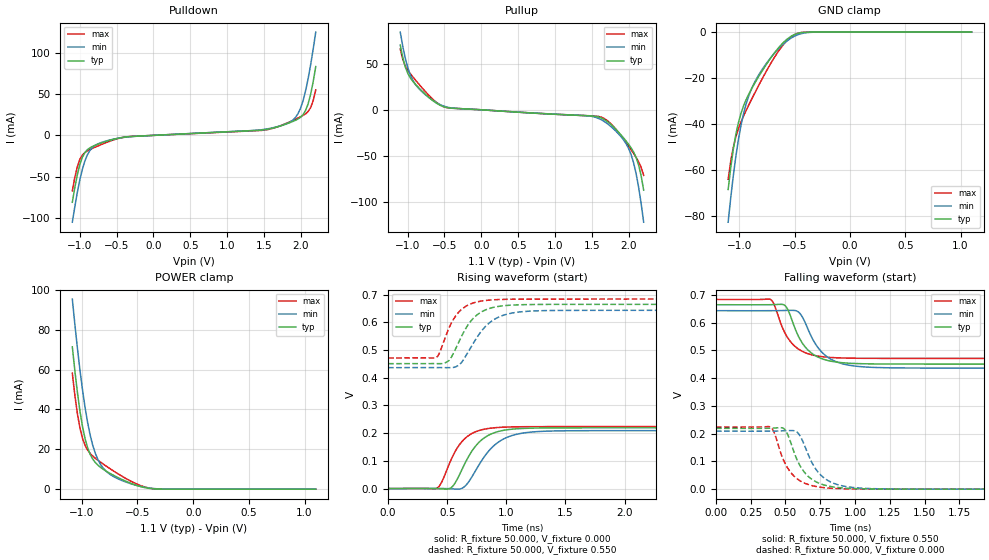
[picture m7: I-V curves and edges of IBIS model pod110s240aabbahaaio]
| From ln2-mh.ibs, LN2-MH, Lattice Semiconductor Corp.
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|   Model pod110s240aabbahaaio
[Model] pod110s240aabbahaaio
| Clamp models do not include dynamic input termination. Please refer to
| the pod110axxxaabbahaain model for input termination.
Model_type I/O
Polarity   Non-Inverting
Enable   Active-Low
Vinl =  0.700V
Vinh =  0.900V
Vmeas =  0.550V
Cref =  20.000pF
Rref =  50.000
Vref =  0.600V
C_comp   2.000pF   1.500pF   2.500pF
[Temperature Range]   25.000   0.125k   -40.000
[Voltage Range]   1.100V   1.070V   1.130V
[C Comp Corner]
C_comp   2.000pF   1.500pF   2.500pF
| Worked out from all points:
|   slope of the pulldown table from 0 to 0.165 V, typ, clamps not added: 226 ohm
|   slope of the pullup table from 0 to 0.165 V, typ, clamps not added: 189 ohm
|   GND clamp passes 1 mA (typ) near -0.50 V on its own axis
|   POWER clamp passes 1 mA (typ) near -0.45 V on its own axis
|   rising waveform, R_fixture 50.000, V_fixture 0.000: 20-80 % time 194ps typ, 223ps min, 170ps max; typ from 0 V to 0.219 V
|   rising waveform, R_fixture 50.000, V_fixture 0.550: 20-80 % time 180ps typ, 213ps min, 152ps max; typ from 0.451 V to 0.665 V
|   falling waveform, R_fixture 50.000, V_fixture 0.550: 20-80 % time 142ps typ, 158ps min, 134ps max; typ from 0.665 V to 0.451 V
|   falling waveform, R_fixture 50.000, V_fixture 0.000: 20-80 % time 136ps typ, 145ps min, 130ps max; typ from 0.219 V to 0 V
[Pulldown]
|Voltage   I(typ)   I(min)   I(max)
-1.1V     -81.17mA   -105.4mA   -67.34mA
-1.032V   -47.86mA   -69.27mA   -37.92mA
-930mV    -20.93mA   -31.09mA   -20.82mA
-862mV    -15.12mA   -18.39mA   -17.27mA
-760mV    -10.94mA   -10.6mA    -13.12mA
-352mV    -1.715mA   -1.886mA   -1.639mA
1.518V    7.039mA    7.489mA    6.6mA
1.892V    16.99mA    18.71mA    18.2mA
1.96V     19.93mA    26.39mA    21.06mA
2.028V    25.15mA    42.13mA    24.19mA
2.13V     49.57mA    85.28mA    33.6mA
2.2V      83.5mA     125.4mA    55.21mA
[Pullup]
|Voltage   I(typ)   I(min)   I(max)
-1.1V     70.38mA    84.41mA    66.13mA
-1.03V    46.02mA    55.41mA    47.25mA
-928mV    30.83mA    31.86mA    35.64mA
-792mV    19.37mA    18.63mA    22.71mA
-554mV    4.731mA    5.428mA    5.061mA
1.452V    -6.529mA   -6.64mA    -6.444mA
1.724V    -13.8mA    -16.09mA   -12.89mA
1.928V    -30.66mA   -32.78mA   -31.94mA
2.03V     -41.41mA   -48.75mA   -43.49mA
2.098V    -51.87mA   -69.53mA   -51.8mA
2.132V    -60.12mA   -84.3mA    -56.57mA
2.2V      -87.31mA   -122.1mA   -71.2mA
[GND_clamp]
|Voltage   I(typ)   I(min)   I(max)
-1.1V     -68.65mA   -82.91mA   -64.16mA
-1.054V   -51.26mA   -62.87mA   -50.37mA
-1.008V   -39.63mA   -47.13mA   -42.26mA
-962mV    -32.34mA   -35.82mA   -36.73mA
-916mV    -27.28mA   -28.13mA   -32.02mA
-847mV    -21.22mA   -20.63mA   -25.4mA
-778mV    -15.81mA   -15.27mA   -19.09mA
-663mV    -7.926mA   -8.201mA   -9.607mA
-571mV    -3.246mA   -3.982mA   -3.828mA
-502mV    -1.097mA   -1.819mA   -1.164mA
-410mV    -96.97uA   -374.9uA   -57.53uA
1.1V      0A         0A         0A
[POWER_clamp]
|Voltage   I(typ)   I(min)   I(max)
-1.085V   71.41mA    95.35mA    58.18mA
-1.062V   59.23mA    82.55mA    46.99mA
-1.039V   48.36mA    70.56mA    37.71mA
-1.016V   38.97mA    59.53mA    30.53mA
-970mV    25.17mA    40.76mA    21.88mA
-924mV    17.37mA    26.93mA    17.87mA
-901mV    15.03mA    21.86mA    16.59mA
-855mV    12.01mA    14.79mA    14.5mA
-763mV    8.448mA    8.108mA    10.89mA
-533mV    2.369mA    2.267mA    3.272mA
-349mV    143.9uA    291.4uA    171.3uA
1.1V      0A         0A         0A
[Ramp]
| variable   typ   min   max
dV/dt_r   0.132/0.194n   0.125/0.224n   0.134/0.171n
dV/dt_f   0.119/0.155n   0.116/0.182n   0.115/0.142n
R_load = 50.000
[Rising Waveform]
R_fixture = 50.000
V_fixture = 0.000
V_fixture_min = 0.000
V_fixture_max = 0.000
|  time   V(typ)   V(min)   V(max)
0s        2.527uV    12.65uV    1.11uV
417ps     24.09uV    252uV      2.484mV
532ps     3.001mV    -643.4uV   103.3mV
621ps     65.34mV    353.3uV    167.8mV
772ps     168.3mV    87.78mV    209.8mV
866ps     195.9mV    142.6mV    217.9mV
962ps     208.9mV    175.6mV    221.3mV
1.157ns   217.3mV    201.4mV    223.2mV
1.507ns   219.1mV    208.5mV    223.6mV
10ns      219.3mV    209.1mV    223.6mV
[Rising Waveform]
R_fixture = 50.000
V_fixture = 0.550
V_fixture_min = 0.534
V_fixture_max = 0.568
|  time   V(typ)   V(min)   V(max)
0s        450.6mV    436.2mV    471.2mV
409ps     450.7mV    436.4mV    473.7mV
510ps     460.3mV    436.2mV    573.9mV
572ps     505mV      439.4mV    623mV
626ps     553.2mV    457.7mV    648mV
722ps     614.9mV    525.2mV    669.9mV
906ps     655.1mV    612.3mV    681.4mV
1.092ns   662.9mV    636.2mV    683.3mV
1.436ns   664.6mV    642.7mV    683.7mV
10ns      664.7mV    643.2mV    683.7mV
[Falling Waveform]
R_fixture = 50.000
V_fixture = 0.550
V_fixture_min = 0.534
V_fixture_max = 0.568
|  time   V(typ)   V(min)   V(max)
0s        664.7mV    643.2mV    683.7mV
392ps     664.8mV    643.2mV    683.7mV
420ps     665.2mV    643.2mV    663.1mV
499ps     660.2mV    644mV      560.1mV
582ps     562.7mV    641.7mV    509mV
651ps     507.1mV    589.2mV    490mV
743ps     473.9mV    504mV      478.8mV
877ps     457.3mV    456.9mV    473.3mV
1.364ns   450.8mV    436.7mV    471.2mV
10ns      450.6mV    436.2mV    471.2mV
[Falling Waveform]
R_fixture = 50.000
V_fixture = 0.000
V_fixture_min = 0.000
V_fixture_max = 0.000
|  time   V(typ)   V(min)   V(max)
0s        219.3mV    209.1mV    223.6mV
391ps     219.8mV    209.1mV    224.1mV
420ps     220.5mV    209.3mV    202.2mV
495ps     214.9mV    210.8mV    94.79mV
573ps     118mV      208.9mV    41.79mV
637ps     60.44mV    157.4mV    21.79mV
723ps     25.59mV    68.87mV    9.278mV
865ps     6.619mV    17.83mV    2.384mV
1.323ns   169.1uV    442.8uV    70.39uV
10ns      2.527uV    12.65uV    1.11uV
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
